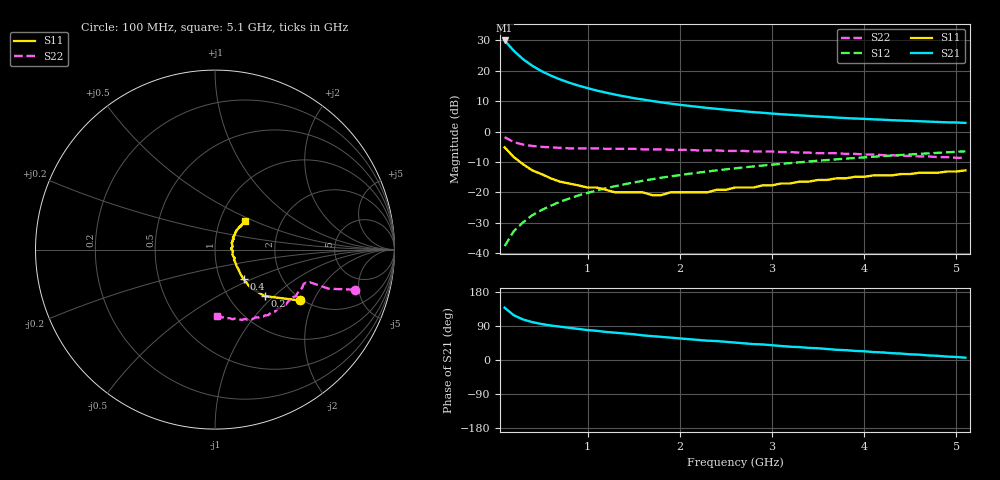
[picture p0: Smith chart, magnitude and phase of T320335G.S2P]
!AT-32033
!S and NOISE PARAMETERS at Vce=5 V  Ic=20mA.  LAST UPDATED 01-05-95
# ghz s ma r 50
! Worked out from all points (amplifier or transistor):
!   51 points, 100 MHz to 5.1 GHz, reference 50 ohm
!   highest |S21| = 30.0 dB at 100 MHz (marker M1)
!   |S21| within 3 dB of that: start of sweep to 187.9 MHz
!   unconditionally stable (mu >= 1): 717.4 MHz to 2.092 GHz; 2.115 GHz to 2.261 GHz
!   at 900 MHz: K = 1.01, MAG = 17.5 dB, |S12| = -21.0 dB
!   at 2.6 GHz: K = 0.99, MSG = 9.5 dB, |S12| = -12.1 dB
!   at 5.1 GHz: K = 0.94, MSG = 4.7 dB, |S12| = -6.5 dB
!   lowest NFmin = 1.38 dB at 500 MHz
!   S11 on the Smith chart (normalised r, x): 100 MHz: 1.94, -1.58; 200 MHz: 1.45, -0.88; 400 MHz: 1.29, -0.45; 5.1 GHz: 1.32, +0.44
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0.1  0.55 -31.0  31.61 138.0  0.013 78.0  0.81 -16.0
0.2  0.38 -43.0  21.34 118.0  0.023 76.0  0.67 -19.0
0.3  0.29 -47.0  15.54 107.0  0.032 77.0  0.61 -19.0
0.4  0.23 -46.0  12.12 100.0  0.042 77.0  0.58 -19.0
0.5  0.2 -44.0  9.9 95.0  0.051 77.0  0.56 -19.0
0.6  0.17 -40.0  8.36 91.0  0.06 77.0  0.55 -20.0
0.7  0.15 -37.0  7.24 88.0  0.07 76.0  0.54 -20.0
0.8  0.14 -34.0  6.39 85.0  0.079 76.0  0.53 -21.0
0.9  0.13 -31.0  5.72 82.0  0.089 75.0  0.53 -22.0
1  0.12 -28.0  5.19 79.0  0.098 74.0  0.53 -23.0
1.1  0.12 -23.0  4.73 77.0  0.107 73.0  0.53 -24.0
1.2  0.11 -21.0  4.38 74.0  0.117 72.0  0.52 -26.0
1.3  0.1 -15.0  4.06 72.0  0.126 71.0  0.52 -27.0
1.6  0.1 -4.0  3.37 65.0  0.155 69.0  0.51 -31.0
1.8  0.09 5.0  3.03 61.0  0.174 66.0  0.51 -33.0
2  0.1 13.0  2.76 57.0  0.192 64.0  0.5 -36.0
2.3  0.1 23.0  2.45 51.0  0.22 61.0  0.49 -40.0
2.6  0.12 29.0  2.22 46.0  0.248 58.0  0.48 -45.0
3.2  0.14 38.0  1.89 35.0  0.303 51.0  0.46 -54.0
3.5  0.16 41.0  1.77 31.0  0.331 48.0  0.44 -59.0
4.3  0.19 43.0  1.54 18.0  0.403 39.0  0.41 -72.0
5.1  0.23 43.0  1.39 6.0  0.473 30.0  0.37 -88.0
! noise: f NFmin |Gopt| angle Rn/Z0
0.5  1.38  0.25  35  0.3
0.9  1.5  0.19  85  0.23
1.8  1.78  0.21  -150  0.14
2.4  1.96  0.39  -114  0.19
